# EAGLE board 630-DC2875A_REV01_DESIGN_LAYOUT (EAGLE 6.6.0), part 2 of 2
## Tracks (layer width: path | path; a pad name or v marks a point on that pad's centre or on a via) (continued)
N$73 (continued)
  Top 0.152: U3.15 84.08,53.59 84.58,53.09 84.58,52.58 85.09,52.07 C9.1 85.81,51.35 87.38,49.78 87.38,46.48 86.87,45.97 84.58,45.97 84.33,46.23 R9.2
N$74  (via drill 0.25)
  Top 0.152: U9.9 104.64,10.42 104.9,10.16 105.41,10.16 | 104.65,7.62 104.39,7.62 104.39,7.58 R57.2 104.43,7.4 104.65,7.62 | 104.65,7.62 105.41,7.62 105.41,10.16 | 105.41,10.16 v108.2,10.16 | v108.2,21.59 102.72,21.59 U8.1
  Route2 0.152: v108.2,10.16 v108.2,21.59
N$75
  Top 0.152: U3.17 84.56,54.59 85.09,55.12 88.9,55.12 89.41,55.63 89.41,56.77 88.39,57.78 88.39,58 R13.1
N$77  (via drill 0.25)
  Top 0.152: U7.8 v84.58,20.7
  Bottom 0.203: v84.58,20.7 86.65,20.7 C47.1
N$78  (via drill 0.25, 0.25 pad 0.25)
  Top 0.152: U3.20 82.01,56.61 82.04,56.64 v82.04,57.66 | RSNS2.1 73.79,65.28 73.53,65.53 NB20.2
  Top 0.203: v82.04,65.02 81.53,65.53 L2.2
  Route2 0.203: v82.04,57.66 v82.04,65.02
  pour Top (no thermals): 74.17,66.29 74.17,64.77 72.39,62.99 72.39,61.85 74.42,61.85 78.61,66.04 82.55,66.04 82.55,67.56 78.11,67.56 76.83,66.29
N$82
  Top 0.152: LED10.2 64.9,44.08 64.9,43.18 65.28,42.8 66.67,42.8 67.31,43.43 M11.5 M11.6
N$83  (via drill 0.25)
  Top 0.152: LED11.3 49.43,46.7 v49.28,46.99
  Route2 0.152: v49.28,46.99 49.28,45.21 v46.74,42.93
  Bottom 0.152: v46.74,42.93 R76.1
N$84
  Top 0.152: M13.5 M13.6 47.37,35.51 47.37,34.92 47.88,34.42 49.53,34.42 50.13,35.02 LED12.2
N$85
  Top 0.152: LED12.4 49.22,35.94 48.51,35.94 48.01,36.45 46.61,36.45 46.1,36.96 46.1,37.61 M13.3
N$86
  Top 0.152: M14.6 M14.5 67.31,34.92 67.18,34.8 65.02,34.8 64.9,34.92 64.9,35.7 LED13.2
N$87
  Top 0.152: LED13.4 64.17,36.35 64.39,36.58 66.29,36.58 66.67,36.96 66.67,37.61 M14.3
N$88  (via drill 0.25)
  Top 0.152: LED13.1 64.87,38.2 65.15,38.48 v65.53,38.48
  Bottom 0.152: v65.53,38.48 R74.1
N$89  (via drill 0.25)
  Top 0.152: v64.26,38.48 64.26,37.52 LED13.3
  Bottom 0.152: R78.1 66.96,37.18 66.8,37.34 66.8,38.1 65.79,39.12 64.9,39.12 v64.26,38.48
N$91  (via drill 0.25)
  Top 0.152: v50.16,38.48 50.16,37.46 LED12.1
  Bottom 0.152: R73.1 48.26,37.72 49.02,38.48 v50.16,38.48
N$92  (via drill 0.25)
  Top 0.152: LED12.3 49.43,38.2 49.15,38.48 v48.13,38.48
  Bottom 0.152: v48.13,38.48 47.5,38.48 46.74,37.72 R77.1
N$94  (via drill 0.25)
  Top 0.152: NB20.1 73.53,67.44 v74.42,68.58 | v87.12,67.82 R15.1
  Route15 0.152: v74.42,68.58 86.36,68.58 v87.12,67.82
N$96
  Top 0.152: LED10.4 64.17,44.73 64.39,44.96 66.29,44.96 66.67,45.34 66.67,45.99 M11.3
N$98
  Top 0.152: R14.1 NB19.1
N$99  (via drill 0.25)
  Top 0.152: NB21.1 72.9,67.56 v73.15,68.07 | v87.12,63.75 R16.1
  Route15 0.152: v73.15,68.07 85.34,68.07 86.36,67.06 86.36,64.52 v87.12,63.75
N$100
  Top 0.152: 80.05,55.88 U3.24
  Top 0.203: U3.26 U3.25 U3.24
  pour Top (no thermals): 80.39,60.96 82.55,60.96 82.55,59.44 81.92,59.44 79.88,57.78 79.88,56.52 80.01,56.39 80.01,55.63 78.99,55.63 78.99,56.39 79.12,56.52 79.12,58.42 80.39,59.44
N$109  (via drill 0.25)
  Top 0.152: NB1.2 45.85,16 v46.1,16.26
  Bottom 0.152: v46.1,16.26 45.85,16.51 R36.1
N$114
  Top 0.203: C10.1 77.47,56.26 77.85,55.88 78.47,55.88 U3.27
N$116
  Top 0.152: U3.12 84.05,52.09 86.36,49.78 R82.2
N$300  (via drill 0.25)
  Top 0.152: NB3.2 v33.78,65.91
  Bottom 0.152: v33.78,65.91 33.53,65.66 33.53,65.15 33.78,64.9 33.78,63.5 34.29,62.99 R22.2
N$301  (via drill 0.25)
  Top 0.152: NB4.2 34.29,66.29 34.54,66.04 34.54,65.53 v34.29,65.28
  Bottom 0.152: v34.29,65.28 34.29,65.02 34.54,64.77 R23.2
N$304  (via drill 0.25)
  Top 0.152: NB7.2 68.07,14.22 v67.56,13.72
  Bottom 0.152: v67.56,13.72 66.67,13.72 66.55,13.59 R47.2
N$305  (via drill 0.25)
  Top 0.152: NB6.2 68.07,14.73 v67.56,15.24
  Bottom 0.152: v67.56,15.24 66.8,15.24 66.67,15.37 R46.2
N$500  (via drill 0.25)
  Top 0.152: NB2.2 46.23,15.49 v46.99,16.26
  Bottom 0.152: v46.99,16.26 47.62,16.26 R37.1
PFET_GATE
  Bottom 0.152: 107.7,39.5 107.7,41.15 107.99,41.44 R29.1 107.95,43.22 107.95,44.2 106.43,44.2 106.43,45.17 R28.2 | 107.7,39.5 107.7,36.32 107.57,36.2 106.76,36.2 M7.1 | M6.1 107.68,39.48 107.7,39.5
PG0
  Top 0.152: U0.G5 58.15,54.85 56.77,53.47 56.77,52.49 R26.1 55.92,52.36 55.37,51.82 55.37,50.04 55.88,49.53 59.94,49.53 60.71,48.77 60.71,47.62 61.47,46.99 | 61.47,46.99 62.36,47.75 66.55,47.75 67.31,46.99 M11.2 | 61.47,46.99 61.47,46.74 | 61.47,46.74 TP16.TP1 | 61.47,46.74 arc-35 61.09,46.1 61.85,46.1 arc-35 61.47,46.74
PG1  (via drill 0.25)
  Top 0.152: U0.G6 59.15,54.83 58.67,54.36 R27.1 59.4,52.36 v59.94,51.82 | v59.94,47.75 52.83,47.75 | M12.2 46.99,47.24 47.5,47.75 52.83,47.75 | 52.83,47.75 52.83,46.86 | 52.83,46.86 52.83,46.74 | 52.83,46.74 TP17.TP1 | 52.83,46.86 arc-35 52.45,46.1 52.58,46.1 | 52.58,46.1 53.09,46.1 | 53.09,46.1 53.21,46.1 arc-35 52.83,46.86 | 52.83,46.74 arc-35 52.58,46.1 | 53.09,46.1 arc-35 52.83,46.74
  Route2 0.152: v59.94,51.82 v59.94,47.75
PG2  (via drill 0.25)
  Top 0.152: M13.2 v46.74,38.48 | U1.G5 58.15,20.3 57.15,19.3 R49.1 56.93,18.33 56.9,18.03 56.39,18.03 56.39,17.27 v55.63,16.51
  Route2 0.152: v55.63,16.51 53.59,16.51 52.07,18.03 52.07,18.8 50.55,20.32 50.55,34.29 51.31,35.05 | 51.31,35.05 TP18.TP1 | 51.31,35.05 arc35 51.82,36.07 51.94,35.94 | 51.94,35.94 52.2,35.69 | 52.2,35.69 52.32,35.56 arc35 51.31,35.05 | 51.31,35.05 arc35 51.94,35.94 | 52.2,35.69 arc35 51.31,35.05
  Route15 0.152: v46.74,38.48 47.24,38.48 49.15,36.58 50.8,36.58 | 50.8,36.58 TP18.TP1 | 50.8,36.58 arc35 51.82,37.08 51.82,36.83 | 51.82,36.83 51.82,36.32 | 51.82,36.32 51.82,36.07 arc35 50.8,36.58 | 50.8,36.58 arc35 51.82,36.83 | 51.82,36.32 arc35 50.8,36.58
PG3  (via drill 0.25)
  Top 0.152: M14.2 v67.31,38.48 | R50.1 59.18,18.29 59.15,18.38 U1.G6 59.15,20.35 59.18,20.32 v61.72,20.32
  Route2 0.152: v61.72,20.32 61.72,21.59 61.09,22.23 61.09,33.66 61.47,34.04 61.47,34.54 | 61.47,34.54 TP19.TP1 | 61.47,34.54 arc35 60.96,35.56 61.16,35.56 | 61.16,35.56 61.77,35.56 | 61.77,35.56 61.98,35.56 arc35 61.47,34.54 | 61.47,34.54 arc35 61.16,35.56 | 61.77,35.56 arc35 61.47,34.54
  Route15 0.152: v67.31,38.48 65.41,36.58 63.5,36.58 | 63.5,36.58 TP19.TP1 | 63.5,36.58 arc-35 62.48,37.08 62.48,36.83 | 62.48,36.83 62.48,36.32 | 62.48,36.32 62.48,36.07 arc-35 63.5,36.58 | 63.5,36.58 arc-35 62.48,36.83 | 62.48,36.32 arc-35 63.5,36.58
PWRGD  (via drill 0.25)
  Top 0.152: U0.G3 56.15,55.39 v55.65,54.86 | U1.G3 56.15,20.84 v55.63,20.32
  Route2 0.152: v55.65,54.86 55.63,53.72 56.01,53.34 56.01,34.42 55.37,33.78 55.37,28.7 55.63,28.19 55.63,24.77 56.26,24.13 56.26,20.92 v55.63,20.32 | v16,63.75 v16,54.86
  Route15 0.152: v16,54.86 v55.65,54.86
  Bottom 0.152: TP4.TP 12.45,63.25 | 12.45,63.25 13.21,63.75 | 13.21,63.75 13.21,64.73 R51.2 | 13.21,63.75 v16,63.75 | 12.45,63.25 arc-35 12.06,62.61 12.83,62.61 arc-35 12.45,63.25
RESETB  (via drill 0.25)
  Top 0.152: v57.67,22.62 57.67,22.61 U1.F5 | U0.F5 58.15,56.37 v57.66,55.92
  Top 0.203: SW1.SW1 19.61,45.51 20.07,45.97 v20.7,45.97
  Route2 0.152: J3.7 104.65,74.68 105.16,74.17 105.16,68.58 v106.93,66.8 106.93,50.04 106.17,49.28 v106.17,48.77 106.17,5.06 J4.7 | v57.67,22.62 58.29,23.24 58.29,27.56 57.78,28.07 57.78,28.7 57.66,28.83 v57.66,48.77 v57.66,55.92
  Route15 0.152: v96.52,67.82 97.54,66.8 v106.93,66.8 | v106.17,48.77 97.92,48.77 97.66,48.51 60.45,48.51 60.2,48.77 v57.66,48.77 23.5,48.77 v20.7,45.97
  Bottom 0.152: RPU2.R3_1 96.16,70.21 96.52,69.85 v96.52,67.82
  Bottom 0.203: v20.7,45.97 21.34,45.97 21.59,45.72 21.59,44.79 C28.2
RUN_CH0  (via drill 0.25)
  Top 0.152: U0.C1 52.59,59.42 v52.58,59.44
  Top 0.203: v77.72,50.8 78.97,50.8 U3.3
  Route2 0.152: v77.98,70.61 77.98,69.34 74.93,66.29 v74.93,60.45 74.93,57.15 76.71,55.37 76.71,51.56 v77.72,50.8
  Route15 0.152: v52.58,59.44 53.59,60.45 55.24,60.45 55.37,60.58 55.88,60.58 56.26,60.2 56.77,60.2 57.28,60.58 64.39,60.58 TP24.1 67.31,60.45 v74.93,60.45
  Bottom 0.152: M1.1 74.79,72.66 75.06,72.39 76.45,72.39 76.96,71.88 77.69,71.88 R63.1 v77.98,70.61
RUN_CH1  (via drill 0.25)
  Top 0.152: U0.B1 52.74,60.42 v52.58,60.58 | U4.5 37.34,53.29 37.34,53.47 v37.97,53.47
  Route2 0.152: v36.83,71.63 36.83,65.28 38.99,63.12 v38.99,58.04 38.99,54.48 v37.97,53.47
  Route15 0.152: v52.58,60.58 46.86,60.58 TP27.1
  Route15 0.203: v38.99,58.04 42.04,58.04 TP27.1
  Bottom 0.152: R64.1 35.6,71.63 v36.83,71.63 37.34,72.14 37.34,73.23 M2.1
RUN_CH2  (via drill 0.25)
  Top 0.152: U1.C1 52.09,25.13 v52.07,25.15 | U6.3 35.66,30.38 v35.56,30.48
  Route2 0.152: TP30.1 v44.96,26.29 44.96,15.24 v40.89,11.18
  Route15 0.152: v52.07,25.15 51.56,25.15 51.44,25.02 50.93,25.02 49.66,26.29 v44.96,26.29 | v40.89,11.18 37.59,11.18 v35.56,9.14 | v35.56,30.48 38.1,27.94 44.2,27.94 TP30.1
  Bottom 0.152: M3.1 40.01,6.15 40.01,5.46 39.75,5.21 37.47,5.21 37.08,5.59 R65.1 37.05,6.35 36.07,6.35 35.56,6.86 v35.56,9.14
RUN_CH3  (via drill 0.25)
  Top 0.152: U1.B1 53.75,26.13 v53.21,26.67 | U7.9 84.08,20.44 83.82,20.7 v83.31,20.7
  Route2 0.152: v53.21,26.67 v53.21,30.48 | TP33.1 64.26,24.89 65.02,24.13 65.02,11.05 66.04,10.03 66.04,6.86 v68.33,4.57 | v83.31,20.7 83.31,9.65 83.06,9.4 v83.06,4.57
  Route15 0.152: v53.21,30.48 58.67,30.48 60.45,28.7 TP33.1 | v68.33,4.57 v75.44,4.57 80.01,4.57 80.52,4.06 82.04,4.06 82.55,4.57 v83.06,4.57
  Bottom 0.152: R66.1 77.07,6.16 M4.1 75.44,6.02 v75.44,4.57
SCL  (via drill 0.25)
  Top 0.152: U1.F7 60.15,22.15 v59.65,22.62 | v59.66,56.92 59.67,56.9 U0.F7 | U8.2 101.67,22.28 v101.6,22.35
  Route2 0.152: v59.66,56.92 59.66,56.24 59.18,55.75 59.18,39.75 59.05,39.62 59.05,39.12 59.18,38.99 59.18,29.46 59.82,28.83 59.82,28.19 59.05,27.43 59.05,23.75 59.66,23.11 v59.65,22.62 58.67,21.59 58.67,19.81 56.39,17.53 v55.63,17.53 | v17.02,16.51 v17.02,29.83
  Route15 0.152: v101.6,22.35 61.21,22.35 60.96,22.61 v59.65,22.62 | v55.63,17.53 54.99,16.89 45.59,16.89 45.21,16.51 v17.02,16.51
  Bottom 0.152: RPU1.R2_1 v17.02,29.83 16.15,29.83 15.49,30.48 14.99,30.48 | 14.99,30.48 TP7.TP | 14.99,30.48 arc-35 14.1,30.99 14.1,30.73 | 14.1,30.73 14.1,30.23 | 14.1,30.23 14.1,29.97 arc-35 14.99,30.48 | 14.1,30.23 arc-35 14.99,30.48 | 14.99,30.48 arc-35 14.1,30.73
SCL_IN  (via drill 0.25)
  Top 0.152: 115.32,41.02 115.32,40.93 R56.2 115.35,40.98 115.32,41.02 | 115.32,41.02 v115.32,41.66 | 103,22.86 102.93,23.06 U8.3 102.5,22.99 v105.16,22.99 | U9.19 103.64,16.5 103.63,16.64 v103.63,17.02
  Route2 0.152: J3.6 102.65,77.69 103.63,76.71 103.63,74.68 104.14,74.17 104.14,67.31 105.92,65.53 105.92,50.29 105.16,49.53 v105.16,42.04 v105.16,22.99 105.16,17.02 | 105.16,17.02 105.16,6.1 103.63,4.57 103.63,2.52 J4.6 | v103.63,17.02 105.16,17.02
  Route15 0.152: J2.4 122.09,41.1 121.16,42.04 115.7,42.04 v115.32,41.66 114.94,42.04 v105.16,42.04
SDA  (via drill 0.25)
  Top 0.152: 59.14,23.12 U1.E6 v58.65,22.63 | v58.66,56.92 58.67,56.94 U0.E6 | v96.52,23.37 96.52,22.23 97.92,22.23 U8.7
  Route2 0.152: v58.66,56.92 58.29,56.52 58.29,28.32 58.67,27.94 58.67,22.86 58.65,22.84 v58.65,22.63 57.66,21.34 57.66,20.32 56.9,19.56 56.39,19.56 v54.36,17.53
  Route15 0.152: v58.65,22.63 59.26,23.24 61.09,23.24 61.47,22.86 65.02,22.86 65.53,23.37 v96.52,23.37 | v54.36,17.53 50.8,17.53 50.55,17.78 v18.54,17.78
  Bottom 0.152: RPU1.R1_1 18.58,21.63 17.27,20.32 | 17.27,20.32 14.99,20.32 | 14.99,20.32 TP8.TP | v18.54,17.78 18.54,19.05 17.27,20.32 | 14.99,20.32 arc-35 14.1,20.83 14.1,20.57 | 14.1,20.57 14.1,20.07 | 14.1,20.07 14.1,19.81 arc-35 14.99,20.32 | 14.99,20.32 arc-35 14.1,20.57 | 14.1,20.07 arc-35 14.99,20.32
SDA_IN  (via drill 0.25)
  Top 0.152: v115.32,43.94 115.32,42.96 R55.2 | U9.20 103.12,16 103.11,15.99 103.12,16.51 v102.62,17.02 102.62,20.07 101.6,21.08 100.84,21.08 98.99,22.93 U8.6
  Route2 0.152: J3.4 100.65,77.66 101.6,76.71 101.6,74.68 103.12,73.15 103.12,67.06 104.14,66.04 v104.14,44.45 104.14,43.94 103.12,42.93 103.12,17.53 v102.62,17.02 103.12,16.51 103.12,5.97 101.73,4.57 101.73,2.62 J4.4
  Route15 0.152: J2.2 122.28,43.32 121.16,44.45 115.82,44.45 v115.32,43.94 114.81,44.45 v104.14,44.45
SGND
  Bottom 0.152: R4.1 C5.2 83.44,41.4 86.87,41.4 R5.1 | 84.52,46.75 U2.37 | 84.09,45.68 U2.37 | 85.86,47.25 85.6,46.99 85.4,46.99 U2.37 | U2.34 84.09,43.95 83.82,43.69 81.53,43.69 80.77,42.93 80.77,40.89 81.06,40.6 R4.1 | 81.79,40.77 81.66,40.64 81.75,40.64 R4.1 | C4.2 90.42,44.2 90.42,43.18 90.17,42.93 90.17,42.42 90.21,42.2 C3.2
  Bottom 0.203: U2.4 84.52,46.75 | U2.34 84.09,45.68 | U2.24 85.86,47.25
  Bottom 0.254: 87.36,47.5 89.41,47.5 90.42,46.48 90.42,44.23 C4.2 | U2.23 87.36,47.5 | 87.36,47.5 U2.24
  pour Bottom (no thermals): 86.87,47.75 87.63,47.75 87.63,47.24 86.36,47.24 86.36,47.37
SHARE_CLK  (via drill 0.25)
  Top 0.152: U1.G4 57.15,20.83 v56.64,20.32 | v56.64,54.86 56.64,54.91 U0.G4 57.15,55.37 v56.64,54.86
  Route2 0.152: v101.09,5.08 101.09,21.97 100.97,22.1 100.97,22.61 101.09,22.73 v101.09,55.24 101.09,65.53 100.33,66.29 100.33,67.56 | 100.33,67.56 TP12.TP | v56.64,20.32 56.64,24.64 56.13,25.15 56.13,29.08 56.77,29.72 56.77,32.38 56.13,33.02 56.13,33.53 56.52,33.91 56.52,54.23 56.64,54.36 v56.64,54.86 | 100.33,67.56 arc35 99.82,68.58 100.08,68.58 | 100.08,68.58 100.58,68.58 | 100.58,68.58 100.84,68.58 arc35 100.33,67.56 | 100.33,67.56 arc35 100.08,68.58 | 100.58,68.58 arc35 100.33,67.56
  Route15 0.152: J4.5 101.11,5.08 v101.09,5.08 | v56.64,54.86 57.02,54.48 59.44,54.48 60.07,53.85 68.33,53.85 69.72,55.24 v101.09,55.24
  Bottom 0.152: RPU2.R2_1 95.23,70.99 96.65,70.99 97.54,70.1 97.79,70.1 | 97.79,70.1 98.04,70.1 | 98.04,70.1 TP12.TP 101.98,71.75 | J3.5 102.65,72.42 102.11,71.88 | 102.11,71.88 101.98,71.75 | 102.11,71.88 arc-35 101.22,71.63 101.35,71.5 | 101.35,71.5 101.73,71.12 | 101.73,71.12 101.85,70.99 arc-35 102.11,71.88 | 97.79,70.1 arc35 98.68,70.61 98.68,70.48 | 98.68,70.48 98.68,69.72 | 98.68,69.72 98.68,69.6 arc35 97.79,70.1 | 98.04,70.1 arc35 98.68,70.48 | 98.68,69.72 arc35 98.04,70.1 | 101.98,71.75 arc-35 101.35,71.5 | 101.73,71.12 arc-35 101.98,71.75
TEMP_CH0  (via drill 0.25)
  Top 0.152: U0.F3 56.15,56.48 v55.65,56.91 | Q1.2 69.29,51.98 C8.1 69.34,52.23 TP25.1
  Route15 0.152: v55.65,56.91 56.01,56.64 57.4,55.24 58.04,55.24 58.17,55.37 60.3,55.37 60.58,55.63 66.04,55.63 TP25.1
TEMP_CH1  (via drill 0.25)
  Top 0.152: U0.F2 v54.65,55.92 | TP28.1 44.96,55.63 44.7,55.24 44.07,55.24 C17.1 43.91,55.37 43.81,55.24 43.65,55.21 Q2.2
  Route15 0.152: v54.65,55.92 54.29,55.92 53.72,56.52 46.61,56.52 TP28.1
TEMP_CH2  (via drill 0.25)
  Top 0.152: U1.F3 56.15,22.11 v55.64,21.64
  Top 0.203: TP31.1 42,28.7 C33.1 41.91,28.07 40.56,28.07 Q3.2
  Route2 0.152: v41.91,19.81 43.18,21.08 43.18,27.69 43.43,27.94 TP31.1
  Route15 0.152: v55.64,21.64 52.58,21.59 50.8,19.81 v41.91,19.81
TEMP_CH3  (via drill 0.25)
  Top 0.152: U1.F2 v55.64,22.61 | Q4.2 90.68,20.03 | 90.68,20.03 92.67,20.03 TP34.1 | C44.1 90.68,20.03
  Route15 0.152: v55.64,22.61 56.39,21.84 66.8,21.84 67.56,21.08 72.39,21.08 73.15,21.84 74.17,21.84 74.42,21.59 85.6,21.59 86.11,21.08 91.69,21.08 TP34.1
UNUSED1
  Route2 0.152: J4.9 106.68,4.33 106.68,4.57 106.93,4.83 106.93,48.26 107.7,49.02 107.7,66.17 110.24,68.71 110.24,72.14 106.66,75.71 J3.9
UNUSED2
  Route2 0.152: J4.10 106.7,1.54 107.7,2.54 107.7,4.06 107.44,4.32 107.44,48.01 108.2,48.77 108.2,65.79 110.74,68.33 110.74,73.53 109.6,74.68 109.6,76.2 109.09,76.71 107.7,76.71 106.7,77.71 J3.10
USB_3.3V  (via drill 0.25)
  Route15 0.152: J2.5 108.73,39.1 v108.71,39.12
  Bottom 0.152: M6.3 108.71,40.07 v108.71,39.12 108.71,37.08 108.65,37.02 M7.3
USB_5V
  Route2 0.406: J3.8 106.44,79.5 112.27,79.5 123.19,68.58 123.19,60.96 120.28,58.05 J2.1
  Bottom 0.254: R60.2 R59.2 114.34,13 C60.1 114.39,11.34 114.55,11.18 115.47,11.18 U10.4
  pour Bottom (no thermals): 120.9,43.69 120.9,42.55 119.38,42.55 118.87,42.04 118.87,19.81 118.11,19.05 118.11,17.78 116.84,16.51 116.84,7.62 111.63,2.41 105.66,2.41 105.28,2.03 105.28,1.02 105.16,0.89 104.14,0.89 104.01,1.02 104.01,2.03 104.65,2.67 111.25,2.67 116.46,7.87 116.46,10.54 116.08,10.92 115.06,10.92 115.06,11.43 116.08,11.43 116.46,11.81 116.46,18.41 118.36,20.32 118.36,42.42 119.63,43.69
VDD33_A  (via drill 0.25)
  Top 0.152: RPU3.R1_2 RPU3.R2_2 RPU3.R3_2 RPU3.R4_2 | R55.1 R56.1 v112.65,40.64 | U0.D2 U0.E2 55.13,57.42 54.63,56.92 53.62,56.92 53.54,56.84 53.14,56.84 53.09,56.9 51.44,56.9 51.18,56.64 51.18,55.66 C30.1 | SW2.SW1 25.65,36.58 | LED8.A LED9.A 29.7,37.08 27.69,37.08 27.18,36.58 25.65,36.58 | U9.18 104.14,16.51 104.39,16.76 v104.39,18.03 | R68.2 v39.12,75.44 | R67.2 v75.18,75.44 | 25.65,36.58 v25.65,35.56
  Top 0.203: 51.18,55.66 50.93,55.5 50.93,54.61 50.16,53.98 v48.26,53.98
  Top 0.254: 98.81,9.11 98.81,7.37 R57.1 | 98.81,9.11 R58.1 | 98.81,9.11 98.81,9.14 97.79,9.14 97.28,9.65 97.28,12.38 RPU3.R1_2 | U8.8 97.98,19.88 98.3,19.56 | C58.1 98.3,19.56 | 98.3,19.56 97.41,18.67 v97.41,18.03 97.41,15.1 RPU3.R4_2
  Route2 0.152: v25.65,35.56 v25.65,42.67
  Route2 0.203: v97.41,18.03 v97.41,28.83 v97.41,40.64 97.41,64.14 v93.34,68.2 | v65.79,46.99 65.79,57.4 v64.52,58.93 v64.52,75.44 | v27.56,73.91 27.56,44.58 v25.65,42.67 | v48.26,46.99 v48.26,53.98 v48.26,75.44
  Route15 0.203: v104.39,18.03 v97.41,18.03 | v112.65,40.64 v104.14,40.64 v97.41,40.64 | v35.56,75.44 29.08,75.44 v27.56,73.91 | v35.56,75.44 v39.12,75.44 v48.26,75.44 | v93.22,75.44 v77.98,75.44 v75.18,75.44 v64.52,75.44 v48.26,75.44 | v48.26,75.44 v35.56,75.44
  Bottom 0.152: R75.2 R71.2 v65.79,46.99 | 48.26,45.72 R72.2 R76.2 48.1,45.56 48.26,45.72 | R52.1 R53.1 102.4,29.12 102.11,28.83 v97.41,28.83 | v104.14,40.64 106.6,40.64 M6.2 | v93.34,68.2 93.34,69.23 RPU2.R4_2 RPU2.R3_2 RPU2.R2_2 RPU2.R1_2 93.26,75.4 v93.22,75.44 | JP1.1 20.54,73.37 20.57,73.41 21.46,73.41 | 21.46,73.41 22.61,73.41 23.11,73.91 25.78,73.91 | 25.78,73.91 v27.56,73.91 27.56,73.03 | 27.56,73.03 27.56,72.78 U11.3 27.62,72.96 27.56,73.03 | U11.1 25.72,73.85 25.78,73.91 | R63.2 v77.98,75.44 | R64.2 v35.56,75.44 | v25.65,42.67 C64.1 | 48.26,45.72 v48.26,46.99 | v64.52,58.93 63.5,58.93 R80.1 | 21.46,73.41 arc-35 20.83,73.79 20.83,73.61 | 20.83,73.61 20.83,73.2 | 20.83,73.2 20.83,73.03 arc-35 21.46,73.41 | 20.83,73.2 arc-35 21.46,73.41 | 21.46,73.41 arc-35 20.83,73.61
  Bottom 0.203: C64.1 25.75,41.15 26.42,41.15 26.67,40.89 27.69,40.89 27.94,41.15 U12.5
VDD33_B  (via drill 0.25)
  Top 0.152: v37.08,9.14 38.73,9.14 39.12,8.76 R69.2 | 75.18,9.14 v77.22,9.14 77.72,9.65 82.3,9.65 82.8,10.16 R41.2 | 75.18,9.14 R70.2 | U1.E2 | U1.E2 U1.D2 | 51.18,21.67 51.26,22.1 C55.1 | U1.E2 55.15,23.61 55.16,23.62 v55.64,23.62 | 75.18,9.14 v75.18,10.92 | 49.49,20.79 49.53,20.83
  Top 0.203: 51.18,21.67 51.18,20.83 | 51.18,20.83 51.69,20.32 52.83,20.32 52.96,20.19 53.47,20.19 53.59,20.32 v54.34,20.32 | 51.18,20.83 49.53,20.83 v48.51,20.83
  Route2 0.152: v55.64,23.62 55.12,23.62 54.86,23.37 54.86,20.84 v54.34,20.32 | v67.06,34.04 v67.06,24.89 v67.06,19.81
  Route2 0.203: v48.51,35.05 v48.51,20.83 48.51,11.3 v47.62,10.41
  Route15 0.152: v37.08,9.14 38.35,10.41 v47.62,10.41 67.06,10.41 67.56,10.92 v75.18,10.92 | v104.39,35.56 95.5,35.56 93.98,34.04 v67.06,34.04 | v67.06,19.81 66.29,19.81 66.04,19.56 55.1,19.56 v54.34,20.32
  Bottom 0.152: R65.2 v37.08,9.14 | R66.2 v77.22,9.14 | R77.2 R73.2 48.51,35.72 v48.51,35.05 | R74.2 R78.2 v67.06,34.04 | v104.39,35.56 104.39,36.32 105.41,37.34 106.6,37.34 M7.2 | v67.06,24.89 63.41,24.89 63.41,25.18 R81.2
VDDIO  (via drill 0.25)
  Top 0.152: R26.2 R27.2 61.18,50.76 v62.23,51.82 | R49.2 R50.2 59.22,16.51 v60.2,16.51 | U1.C7 60.15,25.1 v59.65,24.64 | U0.C7 60.17,59.44 v61.47,59.44
  Route2 0.152: 19.18,71.37 12.95,71.37 10.92,69.34 v10.92,66.55 9.65,65.28 9.65,45.47 v10.16,44.96 9.65,44.45 9.65,35.31 v10.16,34.8 | 19.18,71.37 JP1.2 | v20.32,27.94 v20.32,14.73 | v59.65,24.64 59.66,23.9 60.2,23.37 60.2,22.86 60.25,22.81 60.25,22.35 60.2,22.3 v60.2,16.51 | v62.23,51.82 62.23,58.67 v61.47,59.44 61.98,59.94 61.98,62.36 57.15,67.18 v57.15,76.71 | 19.18,71.37 arc35 20.07,71.75 20.07,70.99 arc35 19.18,71.37
  Route15 0.152: v20.32,14.73 59.18,14.73 60.2,15.75 v60.2,16.51 | v57.15,76.71 25.65,76.71 21.08,72.14 | 21.08,72.14 JP1.2 | 21.08,72.14 arc-35 20.45,71.88 20.83,71.5 arc-35 21.08,72.14
  Bottom 0.152: R51.1 11.65,65.82 v10.92,66.55 | 11.18,44.96 11.38,44.96 M9.1 11.29,45.07 11.18,44.96 | 11.18,44.96 v10.16,44.96 | v10.16,34.8 11.38,34.8 M10.1 11.61,34.8 12.45,34.8 12.95,34.29 19.05,34.29 20.53,32.81 RPU1.R4_2 RPU1.R3_2 RPU1.R2_2 RPU1.R1_2 20.53,28.23 v20.32,27.94
VFB0
  Top 0.152: R10.1 R12.1 R11.1 82.55,49.53 82.51,50 U3.10
VFB1
  Top 0.152: 40.89,59.05 R21.1 | 41.78,59.05 40.89,59.05 | U4.6 37.34,57.49 37.34,58.42 37.97,59.05 40.89,59.05
  Top 0.203: R20.2 R21.1 | R19.1 41.87,59.14 41.78,59.05
VFB2
  Top 0.152: R33.2 R32.1 R31.1 | U6.11 31.11,24 30.1,24 29.46,24.64 R31.1 | R31.1 28.19,24.35 28.19,23.75 27.94,23.5 26.92,23.5 26.67,23.24 26.67,22.39 C37.2
VFB3
  Top 0.152: U7.2 84.07,13.97 84.84,12.95 84.84,12.75 R42.2 R44.2 R45.1
VOUT_CH0  (via drill 0.25)
  Top 0.152: RSNS2.2 72.64,65.28 72.9,65.53 NB21.2 | R12.2 v80.26,45.72
  Route2 0.152: v80.26,45.72 72.14,53.85 72.14,70.1 71.63,70.61 | 71.63,70.61 TP0.TP | 71.63,70.61 arc-35 71.25,71.63 71.12,71.5 | 71.12,71.5 70.74,71.12 | 70.74,71.12 70.61,70.99 arc-35 71.63,70.61 | 70.74,71.12 arc-35 71.63,70.61 | 71.63,70.61 arc-35 71.12,71.5
  Bottom 0.152: 67.56,70.1 64.52,67.06 64.52,65.28 64.55,65.24 R17.2
  Bottom 0.254: 67.94,70.48 arc35 68.33,71.5 68.96,70.87 arc35 67.94,70.48
  Bottom 0.305: RL0.2 67.56,70.1 67.94,70.48 TP0.TP
  pour Top (no thermals): 72.26,64.77 72.26,70.23 70.48,72.14 69.22,72.14 67.44,70.36 62.74,70.36 62.1,70.74 61.21,70.74 61.21,68.07 68.45,68.07 69.85,66.67 70.99,65.41 70.99,64.77
VOUT_CH1  (via drill 0.25)
  Top 0.152: NB4.1 34.29,67.82 34.54,68.07 RSNS3.2 | R21.2 v40.89,65.53
  Route2 0.152: v40.89,65.53 41.78,65.53 44.45,68.2 | 44.45,68.2 44.45,69.85 | 44.45,69.85 TP1.TP | v47.12,65.53 44.45,68.2 | 44.45,69.85 arc-35 44.96,70.87 44.7,70.87 | 44.7,70.87 44.2,70.87 | 44.2,70.87 43.94,70.87 arc-35 44.45,69.85 | 44.2,70.87 arc-35 44.45,69.85 | 44.45,69.85 arc-35 44.7,70.87
  Bottom 0.152: R24.2 v47.12,65.53 | 45.97,71.63 45.21,70.87
  Bottom 0.203: 45.97,71.63 arc35 46.35,70.48 arc35 45.21,70.87
  Bottom 0.406: RL1.2 46.74,70.1 46.35,70.48 TP1.TP
  pour Top (no thermals): 34.92,68.96 40.77,68.96 44.2,72.39 44.96,72.39 46.74,70.36 51.56,70.36 52.32,70.87 53.09,70.87 53.09,68.07 45.97,68.07 44.45,69.47 42.42,67.18 34.92,67.18
VOUT_CH2  (via drill 0.25)
  Top 0.152: NB2.1 44.45,15.49 44.2,15.24 RSNS4.2 | R33.1 v25.4,28.7
  Route2 0.152: v25.4,28.7 24.38,27.69 v24.38,8.13 | TP2.TP 46.1,8.76 | 46.1,8.76 46.23,8.89 | 46.23,8.89 46.48,9.14 46.48,11.18 47.75,12.45 v47.75,25.65 | 46.23,8.89 arc-35 45.21,8.51 45.34,8.38 | 45.34,8.38 45.72,8 | 45.72,8 45.85,7.87 arc-35 46.23,8.89 | 46.1,8.76 arc-35 45.34,8.38 | 45.72,8 arc-35 46.1,8.76
  Route15 0.152: v24.38,8.13 33.78,8.13 34.8,7.11 41.91,7.11 | 41.91,7.11 TP2.TP | 41.91,7.11 arc35 42.93,7.62 42.93,7.37 | 42.93,7.37 42.93,6.86 | 42.93,6.86 42.93,6.6 arc35 41.91,7.11 | 41.91,7.11 arc35 42.93,7.37 | 42.93,6.86 arc35 41.91,7.11
  Bottom 0.152: v47.75,25.65 47.75,26.42 48.26,26.92 R38.2
  Bottom 0.305: 42.42,9.14 arc-35 42.93,7.62 43.94,8.64 arc-35 42.42,9.14
  Bottom 0.406: R35.2 41.4,10.16 42.42,9.14 TP2.TP
  pour Top (no thermals): 43.43,14.86 44.96,14.86 44.96,8.38 45.47,8.13 45.97,8.13 46.74,8.89 50.55,8.89 52.07,10.41 53.09,10.41 53.09,7.87 51.31,7.87 50.55,7.11 43.43,7.11
  pour Bottom (no thermals): 49.66,7.87 49.66,6.35 48.01,6.35 47.12,5.84 45.72,5.84 44.45,7.11 45.97,8.38 47.37,8.38 48.01,7.87
VOUT_CH3  (via drill 0.25)
  Top 0.152: NB7.1 69.34,14.22 69.6,13.97 RSNS5.2 | v88.9,9.14 R45.2
  Route2 0.152: v65.15,27.18 65.15,24.89 65.66,24.38 65.66,11.3 67.94,9.02 | 67.94,9.02 68.2,8.76 | 68.2,8.76 TP3.TP | 67.94,9.02 arc35 69.22,8.51 69.09,8.38 | 69.09,8.38 68.58,7.87 | 68.58,7.87 68.45,7.75 arc35 67.94,9.02 | 68.2,8.76 arc35 69.09,8.38 | 68.58,7.87 arc35 68.2,8.76
  Route15 0.152: TP3.TP 72.39,7.11 | 72.39,7.11 79.5,7.11 80.26,7.87 87.63,7.87 v88.9,9.14 | 72.39,7.11 arc-35 71.37,7.62 71.37,7.37 | 71.37,7.37 71.37,6.86 | 71.37,6.86 71.37,6.6 arc-35 72.39,7.11 | 72.39,7.11 arc-35 71.37,7.37 | 71.37,6.86 arc-35 72.39,7.11
  Bottom 0.152: v65.15,27.18 64.64,27.69 64.14,27.69 63.63,28.19 62.48,28.19 62.48,27.69 62.52,27.65 R48.2
  pour Bottom (no thermals): 64.39,7.87 66.04,7.87 66.67,8.38 68.58,8.38 69.85,7.11 68.58,5.84 66.8,5.84 66.04,6.35 64.39,6.35
  pour Top (no thermals): 68.83,13.46 70.36,13.46 70.36,9.4 70.87,8.89 70.87,7.11 70.36,7.11 66.55,3.3 61.47,3.3 61.21,5.84 66.04,5.84 67.82,7.62 68.83,7.62
VOUT_SNS_CH0  (via drill 0.25)
  Top 0.152: U0.A2 55.15,61.75 55.24,61.85 v55.24,63.88
  Route15 0.152: v55.24,63.88 58.67,63.88 58.8,64.01 59.56,64.01 59.69,63.88 v61.98,63.88
  Bottom 0.152: v61.98,63.88 62.99,63.88 | 62.99,63.88 62.99,63.03 C14.1 | 62.99,63.88 62.99,64.99 R17.1
VOUT_SNS_CH1  (via drill 0.25)
  Top 0.152: v59.18,63.37 59.15,63.34 U0.A6
  Route15 0.152: v59.18,63.37 55.63,63.37 55.5,63.25 54.99,63.25 54.86,63.37 53.72,63.37 v52.83,64.52
  Bottom 0.152: C23.1 R24.1 51.35,64.61 51.44,64.52 v52.83,64.52
VOUT_SNS_CH2  (via drill 0.25)
  Top 0.152: 55.12,27.16 U1.A2 55.15,27.53 54.61,28.07 v54.61,29.21
  Bottom 0.152: v54.61,29.21 52.32,26.92 R38.1 50.29,26.92 50.29,24.64 C41.1
VOUT_SNS_CH3  (via drill 0.25)
  Top 0.152: v59.18,28.45 59.18,27.13 U1.A6
  Bottom 0.152: C52.1 60.96,29.43 60.96,28.45 | 60.96,27.69 60.96,27.43 R48.1 60.92,27.69 60.96,27.69 | 60.96,27.69 60.96,28.45 | 60.96,28.45 v59.18,28.45
VP5P0  (via drill 0.25)
  Top 0.152: U0.G2 55.15,55.4 54.36,54.61 C27.2 54.27,52.32 | 54.99,20.95 54.99,20.97 U1.G2 55.15,21.11 54.99,20.95 | 54.99,20.95 54.99,20.07 52.32,17.4 | 51.05,17.06 C53.1
  Top 0.203: 51.05,17.02 C53.1 51.94,17.02 52.32,17.4 | 54.27,52.32 52.83,52.32 v52.32,51.82 | v51.05,18.54 51.05,17.06
  Route2 0.203: v52.32,51.82 52.32,47.5 51.05,46.23 51.05,37.59 49.78,36.32 49.78,26.29 50.04,26.04 50.04,25.27 49.78,25.02 49.78,19.81 v51.05,18.54
  Route15 0.152: v83.31,31.75 82.04,30.48 v80.77,30.48
  Route15 0.203: v51.05,18.54 66.8,18.54 68.45,20.19 72.26,20.19 73.15,21.08 v73.66,21.08
  Bottom 0.152: U5.4 84.2,32 83.95,31.75 v83.31,31.75 | v80.77,30.48 77.72,30.48
  Bottom 0.203: C26.1 76.45,29.21 73.66,26.42 v73.66,21.08
  Bottom 0.254: 77.72,29.25 C26.1
  Bottom 0.305: L4.2 77.72,30.48 77.72,29.25
VP48V_U0  (via drill 0.25)
  Top 0.152: U0.G1 53.85,55.12 52.7,55.12 v51.56,53.98
  Bottom 0.152: RSNS0.2 74.17,48.51 74.42,48.26 NB13.1 | v51.56,53.98 51.56,50.8 51.31,50.8
  other vias: 75.95,54.48 75.95,53.59 75.18,54.48 75.18,53.59 36.96,49.78 36.96,50.67 39.37,49.78 39.37,50.67
  pour Top (no thermals): 36.83,52.45 36.73,52.7 36.73,53.72 36.93,53.72 36.93,52.7 38.1,51.44 39.37,51.44 39.62,51.18 39.62,49.4 39.37,49.15 36.96,49.15 36.58,49.53 36.58,51.18 36.83,51.44
  pour Bottom (no thermals): 72.39,47.75 73.66,47.75 73.66,50.8 76.45,53.59 76.45,54.86 75.18,54.86 74.93,54.61 74.93,53.34 72.39,50.8 39.88,50.8 39.62,51.05 36.83,51.05 36.58,50.8 36.58,49.53 36.83,49.28 39.62,49.28 39.88,49.53 70.61,49.53
  pour Top (no thermals): 71.88,54.36 71.88,53.34 77.47,53.34 77.47,54.86 74.93,54.86 74.42,54.36
VP48V_U1  (via drill 0.25)
  Top 0.152: U1.G1 53.85,20.83 v53.21,20.83
  Route2 0.152: v53.21,20.83 54.1,21.72 54.1,26.16 53.98,26.29 v53.98,31.11
  Bottom 0.152: v53.98,31.11 54.36,30.73 54.61,30.73
  Bottom 0.203: NB18.1 74.42,39.88 74.17,39.62 RSNS1.2
  other vias: 69.09,33.4 69.98,33.4 69.09,29.59 69.98,29.59 81.66,20.57 80.77,20.57 38.23,32.51 38.23,31.62 38.23,30.73 37.34,30.73
  pour Top (no thermals): 70.36,33.78 70.36,26.92 70.61,26.67 70.61,25.65 68.71,25.65 68.71,29.84 68.83,30.23 68.83,33.78
  pour Bottom (no thermals): 72.64,40.39 73.79,40.39 73.79,37.97 70.36,35.05 70.36,29.21 68.83,29.21 68.83,35.31 72.64,38.61
  pour Route2 (no thermals): 68.83,33.91 70.36,33.91 70.36,28.7 78.11,20.95 82.04,20.95 82.04,19.56 76.96,19.56 68.83,27.69
  pour Top (no thermals): 80.39,20.95 82.04,20.95 82.04,20.57 82.55,20.07 83.57,20.07 83.57,19.18 82.3,19.18 82.04,19.05 80.39,19.05
  pour Top (no thermals): 35.18,32.77 38.61,32.77 38.61,30.73 37.21,29.72 37.21,28.7 36.83,28.7 36.83,30.48 36.2,31.11 35.18,31.11
  pour Bottom (no thermals): 36.83,32.38 36.83,30.35 38.48,30.35 38.86,30.73 67.31,30.73 68.83,29.21 70.36,29.21 70.36,33.78 68.83,33.78 67.31,32.26 39.12,32.26 38.73,32.64 38.1,32.64 37.85,32.38

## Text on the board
tPlace: INSTALL CONNECTORS | ON TOP SIDE | GND | GND | F | E | M | A | L | E | 8-18V | 3.3V | - | + | 1.8V | +32V | +36V | VDDIO | LTC2971 | DAC1 | RUN1 | RUN0 | DAC0 | TMP0 | TMP1 | VDD33 | +48V_EN | RESET | PG1 | PG0 | FAULT | ALERT | LTC2971 | LTC2971 | DEMO CIRCUIT 2875A | FAULT | PG2 | PG3 | High Voltage Power / System Management | TMP2 | RUN2 | RUN3 | DAC3 | LTC2971-1 | DAC2 | RUN | OFF | TMP3 | CONTROL | VDD33 | GND | +24V | -24V | GND | M | A | L | E
bPlace: Rev 1 | A2 | A1 | A0
tStop: LTC2971 | 2-CHANNEL +/-60V | POWER SYSTEM MANAGER | www.analog.com
bStop: POWER SYSTEM MANAGER | 2-CHANNEL +/-60V | LTC2971 | www.analog.com
d_FabDrawing: DRILL TABLE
